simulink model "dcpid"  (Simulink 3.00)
settings: Solver=ode45  StartTime=0.0  StopTime=300  RelTol=1e-6  AbsTol=1e-6
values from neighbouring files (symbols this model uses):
  b = mftrap([-1 4],[1 2])    [example2.m]
undefined symbols (not defined in the file or in its folder): J, K, L, R
libraries: simulink3 x1, simulink_extras x1

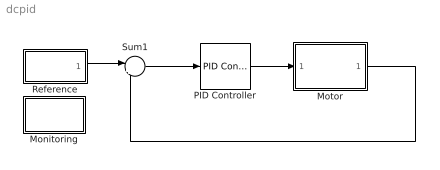
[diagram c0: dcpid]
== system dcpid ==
  Monitoring : Subsystem
  Motor : Subsystem
  PID Controller : simulink_extras/Additional Linear/PID Controller  P=6  I=1  D=0
  Reference : Subsystem
  Sum1 : Sum  Inputs=|+-  SaturateOnIntegerOverflow=on
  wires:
  Sum1/1 -> PID Controller/1
  Reference/1(Out1) -> Sum1/1
  PID Controller/1 -> Motor/1(voltage)
  Motor/1(angle) -> Sum1/2

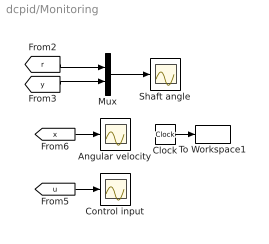
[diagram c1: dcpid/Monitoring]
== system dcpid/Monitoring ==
  Angular velocity : Scope
  Clock : Clock
  Control input : Scope
  Mux : Mux  Inputs=2
  Shaft angle : Scope
  To Workspace1 : ToWorkspace  VariableName=t  SampleTime=0.1  SaveFormat=Matrix
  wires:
  [y] -> Mux/2
  [r] -> Mux/1
  Mux/1 -> Shaft angle/1
  [u] -> Control input/1
  Clock/1 -> To Workspace1/1
  [x] -> Angular velocity/1

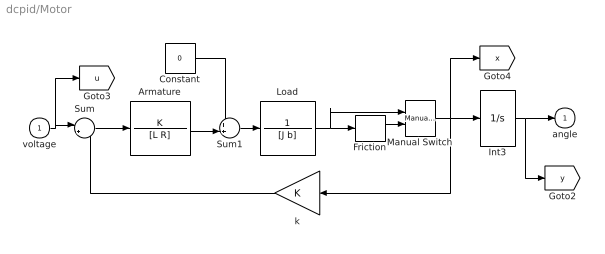
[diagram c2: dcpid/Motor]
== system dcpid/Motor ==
  voltage : Inport  Port=1  PortWidth=-1  SampleTime=-1  DataType=auto
  " k " : Gain  Orientation=left  Gain=K  SaturateOnIntegerOverflow=on
  Armature : TransferFcn  Numerator=K  Denominator=[L R]
  Constant : Constant  Value=0
  Friction : DeadZone  LowerValue=-0.005  UpperValue=0.01
  Int3 : Integrator  ExternalReset=none  InitialConditionSource=internal  InitialCondition=.1  LimitOutput=off  UpperSaturationLimit=inf  LowerSaturationLimit=-inf  ShowSaturationPort=off  ShowStatePort=off  AbsoluteTolerance=auto
  Load : TransferFcn  Numerator=1  Denominator=[J b]
  Manual Switch : simulink3/Nonlinear/Manual Switch  sw=1  action=0
  Sum : Sum  Inputs=|+-  SaturateOnIntegerOverflow=on
  Sum1 : Sum  Inputs=++|  SaturateOnIntegerOverflow=on
  angle : Outport  Port=1
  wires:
  Sum/1 -> Armature/1
  voltage/1 -> Sum/1, [u]
  Armature/1 -> Sum1/2
  " k "/1 -> Sum/2
  Friction/1 -> Manual Switch/2
  Manual Switch/1 -> Int3/1, " k "/1, [x]
  Load/1 -> Friction/1, Manual Switch/1
  Int3/1 -> angle/1, [y]
  Sum1/1 -> Load/1
  Constant/1 -> Sum1/1

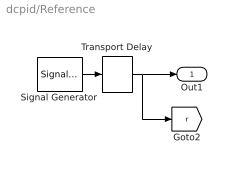
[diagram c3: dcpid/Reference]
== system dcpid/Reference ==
  Signal Generator : SignalGenerator  WaveForm=square  Amplitude=0.100000  Frequency=1/200  Units=Hertz
  Transport Delay : TransportDelay  DelayTime=50  InitialInput=0  BufferSize=1024
  Out1 : Outport  Port=1
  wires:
  Signal Generator/1 -> Transport Delay/1
  Transport Delay/1 -> Out1/1, [r]
